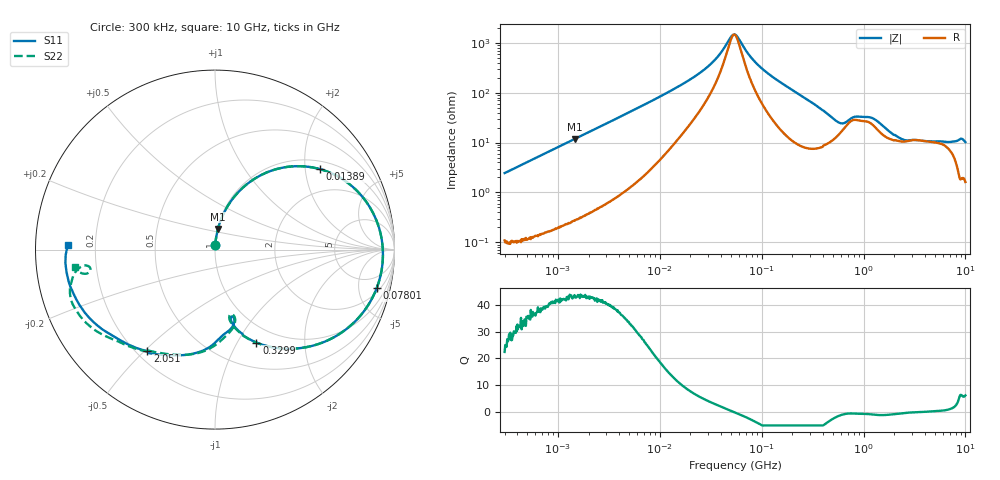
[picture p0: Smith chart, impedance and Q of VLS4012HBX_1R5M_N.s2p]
! S-Parameter Data Generated by TDK Corporation
! Copyright(C) 2023 TDK Corporation.
! All Rights Reserved.
! TDK P/N: VLS4012HBX-1R5M-N (Inductor)
! Property: L=1.5uH at 1MHz
! Size(LxWxT): 4x4x1.2mm
! Model Type: s2p (Touchstone File Format Version 1.0)
! Frequency: DC=Yes Start=0.3MHz Stop=10000MHz 802points Log-sweep
! Model Generated on June 16, 2023
! Port Assignments:
!  1 ---@@@--- 2
! Applicable Conditions:
!  Temperature = 25 degC
!  DC Bias Current = 0 A
!  Small Signal Operation
! Terms and conditions regarding TDK Simulation Models
! (1)This simulation model is being provided solely for informational purposes. Please refer to the specifications of the products in terms of detailed characteristics of such products.
! (2)In no event shall TDK Corporation of any of its subsidiaries be liable for any loss or damage arising, directly or indirectly,
!  From any information contained in this simulation model, including, but not limited to loss or damages arising from any inaccuracies, omissions or errors in connection with such information.
! (3)Any and all copyrights on this simulation model are owned by TDK Corporation.
!  Duplication or redistribution of this simulation model without prior written permission from TDK Corporation is prohibited.
! (4)This simulation model is subject to any modification or change without any prior notice.
! (5)Neither TDK Corporation nor any of its subsidiaries shall make any warranty, express or implied,
!  Including but not limited to the correctness, implied warranties of merchantability and fitness for a particular purpose with respect to this simulation models.
! (6)The use of this simulation model shall be deemed to have consented to the terms and conditions hereof.
# Hz S MA R 50
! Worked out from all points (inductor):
!   801 points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, 300 kHz to 10 GHz, reference 50 ohm
!   read as one part in series: L = 1.29 uH near 318.3 kHz
!   highest Q = 43.4 at 1.457 MHz (marker M1), where L = 1.28 uH
!   self-resonance near 53.76 MHz
!   S11 on the Smith chart (normalised r, x): 300 kHz: 1.00, +0.05; 13.89 MHz: 1.22, +2.40; 78.01 MHz: 2.54, -7.68; 329.9 MHz: 0.79, -1.21; 2.051 GHz: 0.24, -0.51; 10 GHz: 0.10, +0.02
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300000  0.02417 86.0  0.9985 -1.4  0.9987 -1.4  0.02392 86.0
1456635  0.1159 82.0  0.9905 -6.7  0.9907 -6.7  0.1158 81.9
1713600  0.1357 80.8  0.9875 -7.9  0.9877 -7.9  0.1358 80.8
4549142  0.34 68.3  0.9306 -20.1  0.9309 -20.1  0.34 68.3
9671944  0.6088 49.1  0.7624 -37.9  0.7624 -37.9  0.6088 49.1
1.388558e7  0.7371 37.5  0.6195 -48.0  0.6196 -48.0  0.7371 37.5
2.987769e7  0.9017 13.6  0.2678 -62.6  0.2679 -62.6  0.9018 13.6
5.477226e7  0.9365 -3.2  0.06399 4.2  0.064 4.2  0.9365 -3.2
7.800823e7  0.9262 -13.4  0.1764 56.7  0.1764 56.7  0.9262 -13.4
1.063884e8  0.8944 -23.4  0.316 56.4  0.3161 56.4  0.8943 -23.4
1.69821e8  0.794 -40.6  0.5347 43.8  0.5348 43.8  0.7938 -40.5
3.126428e8  0.5866 -64.1  0.7538 20.3  0.7539 20.3  0.5859 -64.2
3.29906e8  0.5671 -65.9  0.7662 18.1  0.7664 18.1  0.5663 -66.1
4.866838e8  0.4365 -76.1  0.8109 1.7  0.811 1.7  0.4331 -76.9
6.656121e8  0.386 -75.3  0.7643 -12.1  0.7644 -12.1  0.3711 -75.7
1.001841e9  0.4844 -85.6  0.6737 -20.8  0.6738 -20.8  0.497 -84.7
1.767019e9  0.6531 -116.0  0.6294 -37.9  0.6295 -37.9  0.6554 -118.9
2.051294e9  0.6807 -123.7  0.6032 -44.2  0.6033 -44.2  0.6871 -124.6
4.516006e9  0.8108 -156.2  0.3672 -78.0  0.3672 -78.0  0.8259 -150.4
6.899057e9  0.8353 -169.3  0.2795 -95.3  0.2796 -95.4  0.8449 -162.8
8.322921e9  0.8332 -177.3  0.2393 -106.3  0.2394 -106.4  0.751 -172.8
1e10  0.82 178.2  0.2271 -111.0  0.2273 -111.1  0.7871 -172.9
